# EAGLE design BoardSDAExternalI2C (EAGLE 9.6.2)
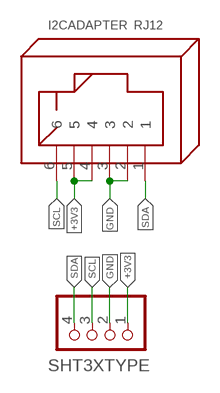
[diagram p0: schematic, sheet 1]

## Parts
I2CADAPTER  RJ12  [RJ12]
SHT3XTYPE  PINHD-1X4  [1X04]

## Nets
+3V3: I2CADAPTER.4 I2CADAPTER.5 SHT3XTYPE.1
GND: I2CADAPTER.2 I2CADAPTER.3 SHT3XTYPE.2
SCL: I2CADAPTER.6 SHT3XTYPE.3
SDA: I2CADAPTER.1 SHT3XTYPE.4

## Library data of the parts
I2CADAPTER = con-rj:RJ12: RJ12, RJ14 and RJ25 RJ12, RJ14 and RJ25 jacks side mounted http://www.tycoelectronics.com
SHT3XTYPE = pinhead:PINHD-1X4: PIN HEADER

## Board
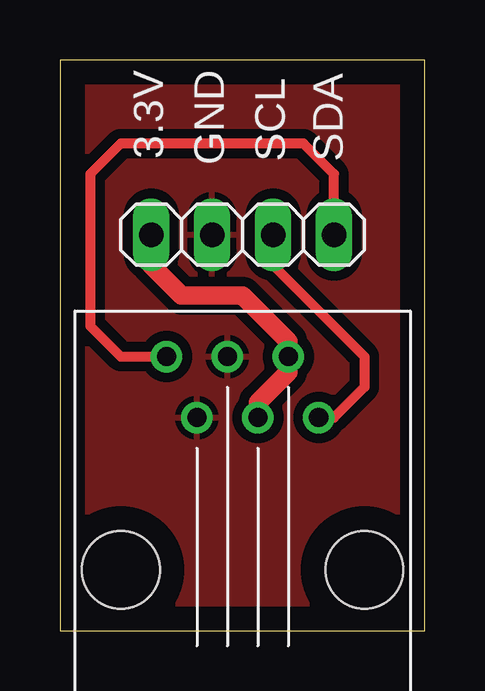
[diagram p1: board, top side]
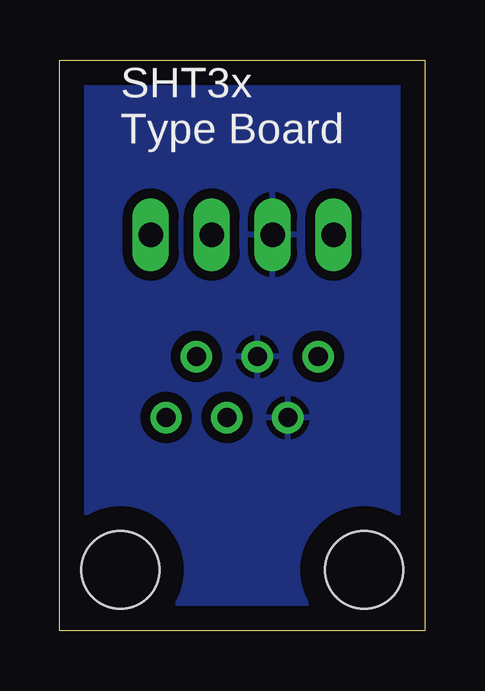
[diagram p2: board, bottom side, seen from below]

Size 15.22 x 23.8 mm. Coordinates in mm from the lower left corner, seen from the top.
Outline: 0,0 15.22,0 15.22,23.8 0,23.8 0,0
Copper layers (1*16): Top 0.035mm / dielectric 1.5mm / Bottom 0.035mm
Design rules "default": minimum track width 6mil, minimum drill 0.35mm, track to track 6mil, track to pad 6mil, pad to pad 6mil, via to via 6mil, smd to smd 6mil, copper to edge 40mil, drill to drill 6mil, minimum pad ring 10mil, minimum via ring 8mil, stop-mask expansion 4mil, vias tented up to drill 0mil, thermal gap 10mil

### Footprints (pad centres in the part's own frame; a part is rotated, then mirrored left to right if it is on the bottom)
RJ12 = drill 0.8: 1 -8.89,-3.175; 2 -6.35,-1.905; 3 -8.89,-0.635; 4 -6.35,0.635; 5 -8.89,1.905; 6 -6.35,3.175 | hole 3.25: 0,-5.08; 0,5.08
1X04 = drill 1.016 long: 1 -3.81,0; 2 -1.27,0; 3 1.27,0; 4 3.81,0

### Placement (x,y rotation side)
I2CADAPTER  7.62,2.54 270 top
SHT3XTYPE  7.62,16.51 0 top

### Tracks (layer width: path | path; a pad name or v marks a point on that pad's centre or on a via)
+3V3
  Top 0.762: I2CADAPTER.4 8.26,9.53 9.53,10.79 I2CADAPTER.5 9.53,12.06 7.62,13.97 5.08,13.97 3.81,15.24 SHT3XTYPE.1
GND
  pour Top (isolate 0.406): 0,24.13 15.24,24.13 15.24,0 0,0
  pour Bottom (isolate 0.406): 0,24.13 15.24,24.13 15.24,0 0,0
SCL
  Top 0.406: SHT3XTYPE.3 8.89,15.24 12.7,11.43 12.7,10.16 11.43,8.89 I2CADAPTER.6
SDA
  Top 0.406: SHT3XTYPE.4 11.43,19.05 10.16,20.32 2.54,20.32 1.27,19.05 1.27,12.7 2.54,11.43 I2CADAPTER.1

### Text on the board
tPlace: 3.3V | SCL | SDA | GND
bPlace: SHT3x / Type Board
